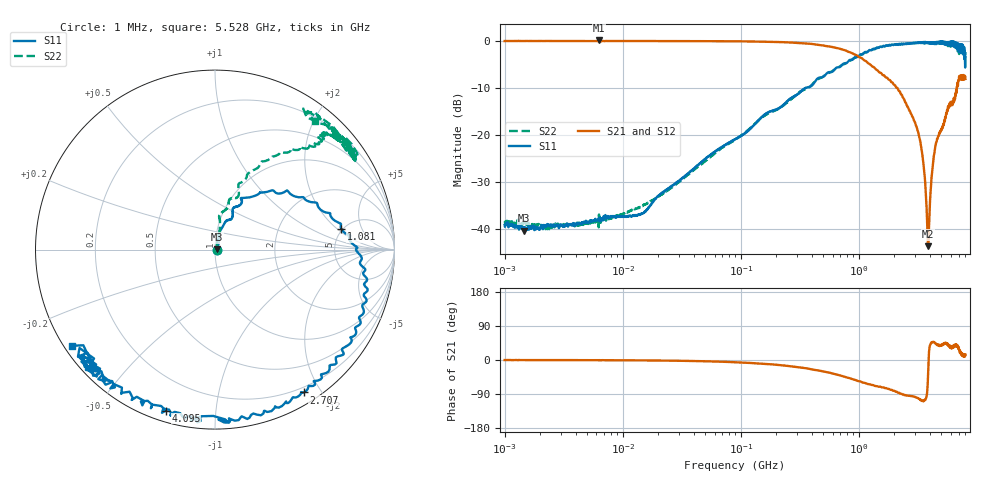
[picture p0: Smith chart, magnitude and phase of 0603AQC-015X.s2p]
!s-Parameter Generated by FASTRON Sdn. Bhd.
!FASTRON P/N : 0603AQC-015X
!Keysight Technologies: E5071C_MY46733604_B.14.02
!Date: Thu Jun 25 13:51:56 2026
!Version  :Rev00  Thu Jun 25 13:51:56 2026
!Data & Calibration Information:
!Freq  S11:SOLT2(ON)  S21:SOLT2(ON)  S12:SOLT2(ON)  S22:SOLT2(ON)
!PortZ  Port1:50+j0  Port2:50+j0
!When reading reference impedance value at option line is always used.
! Remarks : This data is being provided solely for informational purposes.
# Hz S dB R 50
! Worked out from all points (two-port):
!   1601 points, 1 MHz to 8 GHz, reference 50 ohm
!   highest |S21| = 0.02 dB at 6.301 MHz (marker M1); lowest = -43.6 dB at 3.872 GHz (marker M2)
!   |S21| within 3 dB of the highest: start of sweep to 924.8 MHz
!   lowest |S11| = -40.3 dB at 1.459 MHz (marker M3), VSWR 1.02, Z = 51 + j0.0756 ohm
!   |S11| at or under -10 dB: start of sweep to 357.9 MHz
!   |S22| runs from -40.0 to -0.3 dB; largest |S21 - S12| = 0.0099
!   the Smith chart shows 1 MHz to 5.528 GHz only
!   S11 on the Smith chart (normalised r, x): 1 MHz: 1.02, +0.00; 1.081 GHz: 4.90, +2.27; 2.707 GHz: 0.14, -1.79; 4.095 GHz: 0.05, -0.74; 5.528 GHz: 0.02, -0.31
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1000000  -39.10 1.8  -0.11 -0.1  -0.11 -0.0  -38.30 2.6
1459186  -40.30 4.4  -0.10 -0.2  -0.11 -0.1  -38.80 -2.4
4479405  -38.60 20.8  -0.10 -0.4  -0.11 -0.3  -38.80 24.6
6301378  -37.70 31.5  0.02 -0.3  0.01 -0.2  -36.90 28.1
1.449233e7  -36.60 44.5  -0.10 -1.0  -0.12 -1.1  -35.10 47.5
2.00676e7  -32.90 50.7  -0.11 -1.4  -0.12 -1.3  -33.10 61.9
8.994653e7  -20.90 76.8  -0.16 -5.9  -0.17 -5.9  -21.00 74.4
4.006501e8  -9.55 59.9  -0.72 -24.7  -0.73 -24.7  -9.37 66.9
6.624464e8  -5.67 39.0  -1.63 -39.0  -1.63 -39.0  -5.80 62.5
1.080879e9  -2.93 9.2  -3.93 -59.5  -3.94 -59.6  -2.80 50.1
1.7949e9  -0.99 -21.9  -8.30 -76.3  -8.33 -76.5  -0.99 46.4
2.706981e9  -0.57 -58.2  -14.90 -94.6  -15.00 -94.5  -0.62 45.0
3.345355e9  -0.47 -81.4  -21.90 -106.0  -21.90 -106.0  -0.48 39.8
3.872345e9  -0.40 -100.0  -43.60 -25.0  -43.70 -26.3  -0.49 40.4
4.095302e9  -0.56 -107.0  -30.60 45.8  -30.60 45.4  -0.53 45.6
4.520586e9  -0.56 -127.0  -21.60 41.7  -21.60 41.4  -0.76 37.2
4.912472e9  -0.59 -136.0  -19.10 37.9  -19.10 37.7  -0.69 35.7
5.528293e9  -0.37 -146.0  -15.60 42.0  -15.60 41.8  -0.83 52.0
6.110812e9  -0.50 -164.0  -13.40 30.0  -13.30 29.6  -1.03 43.8
6.920464e9  -0.58 -173.0  -9.52 34.7  -9.50 34.0  -1.44 70.5
7.498787e9  -0.81 153.0  -8.34 11.8  -8.36 11.0  -1.63 55.2
8e9  -3.51 144.0  -8.14 14.5  -8.16 13.7  -2.44 61.8
